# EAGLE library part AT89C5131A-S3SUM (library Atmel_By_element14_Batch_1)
8-bit Flash Microcontroller
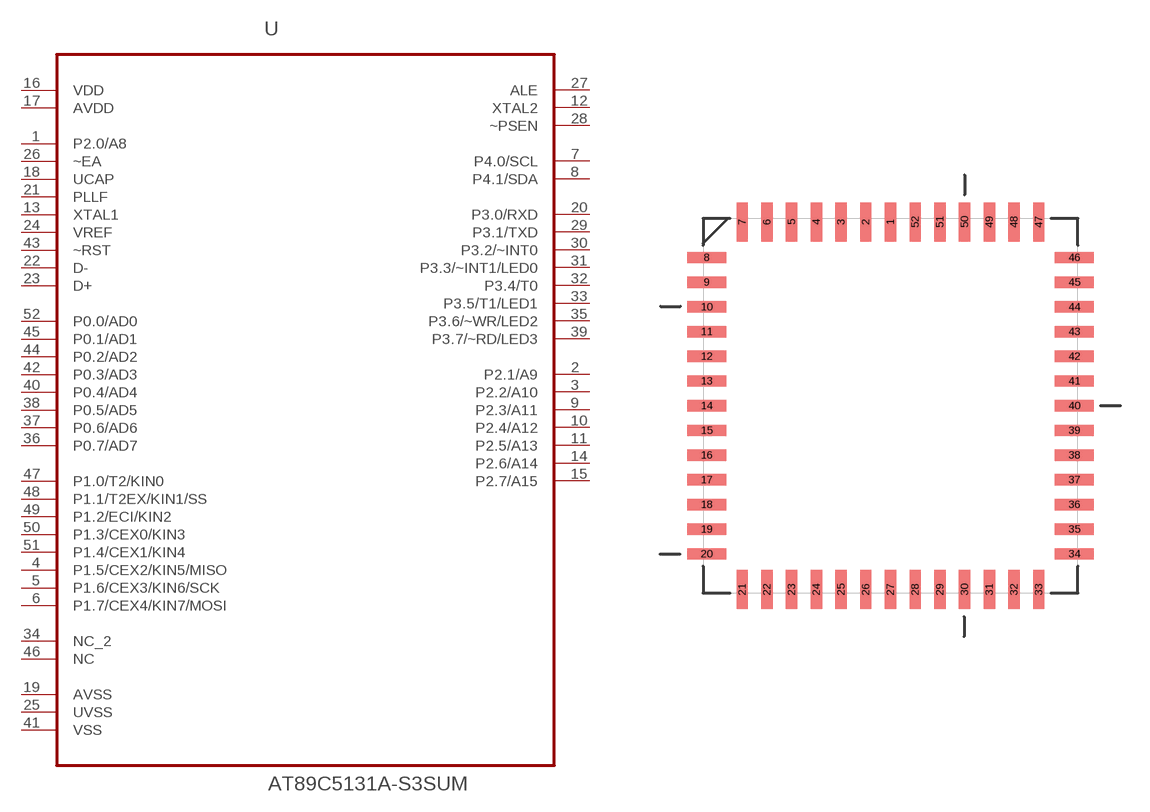
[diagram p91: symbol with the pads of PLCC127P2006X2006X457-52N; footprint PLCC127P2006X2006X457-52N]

Designator prefix U

## AT89C5131A-S3SUM (DESCRIPTION: 8-bit Flash Microcontroller; MPN: AT89C5131A-S3SUM; OC_FARNELL: 1095721; OC_NEWARK: 96K6570; PACKAGE: PLCC-52; SUPPLIER: Atmel)  [PLCC127P2006X2006X457-52N]
1  P2.0/A8
2  P2.1/A9
3  P2.2/A10
4  P1.5/CEX2/KIN5/MISO
5  P1.6/CEX3/KIN6/SCK
6  P1.7/CEX4/KIN7/MOSI
7  P4.0/SCL
8  P4.1/SDA
9  P2.3/A11
10  P2.4/A12
11  P2.5/A13
12  XTAL2  out
13  XTAL1  in
14  P2.6/A14
15  P2.7/A15
16  VDD  pwr
17  AVDD  pwr
18  UCAP  pas
19  AVSS  pwr
20  P3.0/RXD
21  PLLF  pas
22  D-  pas
23  D+  pas
24  VREF  in
25  UVSS  pwr
26  ~EA  in
27  ALE  out
28  ~PSEN  out
29  P3.1/TXD
30  P3.2/~INT0
31  P3.3/~INT1/LED0
32  P3.4/T0
33  P3.5/T1/LED1
34  NC_2  nc
35  P3.6/~WR/LED2
36  P0.7/AD7
37  P0.6/AD6
38  P0.5/AD5
39  P3.7/~RD/LED3
40  P0.4/AD4
41  VSS  pwr
42  P0.3/AD3
43  ~RST  in
44  P0.2/AD2
45  P0.1/AD1
46  NC  nc
47  P1.0/T2/KIN0
48  P1.1/T2EX/KIN1/SS
49  P1.2/ECI/KIN2
50  P1.3/CEX0/KIN3
51  P1.4/CEX1/KIN4
52  P0.0/AD0

## Footprint PLCC127P2006X2006X457-52N (pad centres in mm)
smd 0.584 x 2.007: 1 0,9.449; 2 -1.27,9.449; 3 -2.54,9.449; 4 -3.81,9.449; 5 -5.08,9.449; 6 -6.35,9.449; 7 -7.62,9.449; 21 -7.62,-9.449; 22 -6.35,-9.449; 23 -5.08,-9.449; 24 -3.81,-9.449; 25 -2.54,-9.449; 26 -1.27,-9.449; 27 0,-9.449; 28 1.27,-9.449; 29 2.54,-9.449; 30 3.81,-9.449; 31 5.08,-9.449; 32 6.35,-9.449; 33 7.62,-9.449; 47 7.62,9.449; 48 6.35,9.449; 49 5.08,9.449; 50 3.81,9.449; 51 2.54,9.449; 52 1.27,9.449
smd 2.007 x 0.584: 8 -9.449,7.62; 9 -9.449,6.35; 10 -9.449,5.08; 11 -9.449,3.81; 12 -9.449,2.54; 13 -9.449,1.27; 14 -9.449,0; 15 -9.449,-1.27; 16 -9.449,-2.54; 17 -9.449,-3.81; 18 -9.449,-5.08; 19 -9.449,-6.35; 20 -9.449,-7.62; 34 9.449,-7.62; 35 9.449,-6.35; 36 9.449,-5.08; 37 9.449,-3.81; 38 9.449,-2.54; 39 9.449,-1.27; 40 9.449,0; 41 9.449,1.27; 42 9.449,2.54; 43 9.449,3.81; 44 9.449,5.08; 45 9.449,6.35; 46 9.449,7.62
